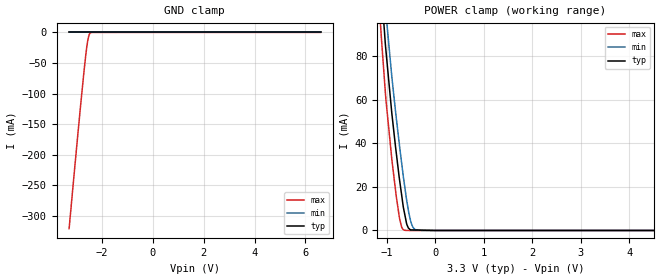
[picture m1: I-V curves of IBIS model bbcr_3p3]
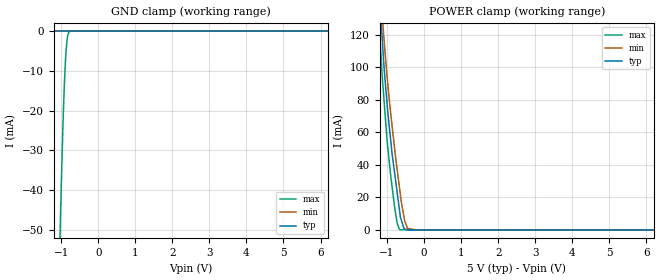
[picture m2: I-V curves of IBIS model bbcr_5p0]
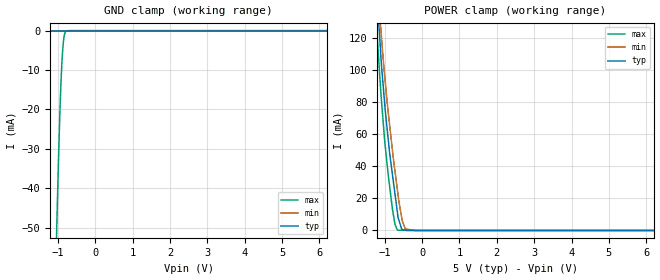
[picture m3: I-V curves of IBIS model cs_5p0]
|Texas Instruments Incorporated
|18 Bit 500KSPS Parallel ADC
| Marketing part#   Digital Voltage Range   Package-type   #pins
| ADS8383IBPFBT   2.95V - 5.25V   TQFP   48
| ADS8383IBPFBTG4   2.95V - 5.25V   TQFP   48
| ADS8383IPFBT   2.95V - 5.25V   TQFP   48
| ADS8383IPFBTG4   2.95V - 5.25V   TQFP   48
[IBIS Ver]   3.2
[File name]   ads8383.ibs
|SIMDE Ver   V3.0 - 201101 - RHL4 - Build 457
[File Rev]   1.1
[Date]   11/11/2011
[Source]
| Texas Instruments Incorporated.
| Analog-eLab Design Center, HPA
| 12500 TI Blvd
| Dallas, TX -75243
| e-mail: elab_scm_ibis@list.ti.com
[Notes]   Revision History:
| Rev 1.1: 11/11/2011
| - Model generated from simulations in TISPICE
| - Model matched to SPICE simulation
| - C_comp although listed in numerical order of value are
|   obtained from varying PVT conditions. For PVT conditions for
|   each specific value refer the buffer description under
|   respective [Model]. IBIS model user is responsible for using
|   appropriate C_comp to simulate for Signal Integrity.
| - Model names with a trailing _5 contains the model for
|   5V [4.75V and 5.25V].
| - Model names with a trailing _3p3 contains the model for
|   3.3V [3V and 3.6V].
[Disclaimer]
| This model is designed as an aid for customers of Texas Instruments.
| TI and its licensors and suppliers make no warranties, either expressed
| or implied, with respect to this  model, including the warranties of
| merchantability or fitness for a particular purpose. The model is
| provided solely on an "as is" basis. The entire risk as to its quality
| and performance is with the customer.
[Copyright]
 (C) Copyright 2011 Texas Instruments Incorporated.All rights reserved.
|   ADS8383PFB
[Component]   ADS8383PFB
[Manufacturer]   TI
[Package]   |48 TQFP  -  PFB package
|   typ   min   max
R_pkg   0.087796   0.08287   0.10031
L_pkg   2.915612nH   2.61503nH   3.79551nH
C_pkg   0.471017pF   0.40218pF   0.58411pF
[Pin]  signal_name   model_name   R_pin   L_pin   C_pin
1   REFIN   TERM   0.10010   3.79551nH  0.57733pF
2   NC   NC   0.09197   3.05397nH  0.50922pF
3   NC   NC   0.08751   2.91787nH  0.48805pF
4   +VA   POWER   0.08536   2.88283nH  0.48088pF
5   AGND   GND   0.08494   2.68463nH  0.43457pF
6   +IN   TERM   0.08529   2.66218nH  0.40388pF
7   -IN   TERM   0.08477   2.65050nH  0.40398pF
8   AGND   GND   0.08402   2.66577nH  0.43614pF
9   +VA   POWER   0.08491   2.87617nH  0.48351pF
10   +VA   POWER   0.08836   2.93642nH  0.49009pF
11   AGND   GND   0.09080   3.03060nH  0.51172pF
12   AGND   GND   0.10050   3.79783nH  0.58722pF
13   +VA   POWER   0.09984   3.80136nH  0.57430pF
14   AGND   GND   0.09184   3.06007nH  0.50608pF
15   AGND   GND   0.08798   2.93541nH  0.48558pF
16   DB17   DB   0.08570   2.89372nH  0.48372pF
17   DB16   DB   0.08388   2.66997nH  0.43641pF
18   DB15   DB   0.08343   2.63103nH  0.40274pF
19   DB14   DB   0.08310   2.62211nH  0.40279pF
20   DB13   DB   0.08287   2.64801nH  0.43550pF
21   DB12   DB   0.08400   2.86018nH  0.48130pF
22   DB11   DB   0.08636   2.90203nH  0.48479pF
23   DB10   DB   0.09049   3.02875nH  0.50816pF
24   +VBD   POWER   0.09815   3.75628nH  0.57908pF
25   BDGND   GND   0.09823   3.76461nH  0.57325pF
26   DB9   DB   0.09338   3.08747nH  0.50871pF
27   DB8   DB   0.08903   2.95227nH  0.48968pF
28   DB7   DB   0.08642   2.90683nH  0.48351pF
29   DB6   DB   0.08500   2.68753nH  0.43735pF
30   DB5   DB   0.08491   2.65538nH  0.40456pF
31   DB4   DB   0.08489   2.65260nH  0.40489pF
32   DB3   DB   0.08497   2.68317nH  0.43773pF
33   DB2   DB   0.08639   2.90287nH  0.48281pF
34   DB1   DB   0.08893   2.94342nH  0.48973pF
35   DB0   DB   0.09324   3.07400nH  0.51329pF
36   BUSY   BUSY   0.10031   3.78743nH  0.58411pF
37   +VBD   POWER   0.09816   3.75870nH  0.57356pF
38   BUS18/_16   BBCR   0.09050   3.02494nH  0.50569pF
39   BYTE   BBCR   0.08638   2.89432nH  0.48541pF
40   _CONVST   BBCR   0.08400   2.85234nH  0.48080pF
41   _RD   BBCR   0.08288   2.64046nH  0.43471pF
42   _CS   CS   0.08311   2.61503nH  0.40218pF
43   +VA   POWER   0.08344   2.61976nH  0.40287pF
44   AGND   GND   0.08386   2.65850nH  0.43615pF
45   AGND   GND   0.08552   2.88190nH  0.48159pF
46   +VA   POWER   0.08742   2.91318nH  0.48615pF
47   REFM   TERM   0.09183   3.04637nH  0.51100pF
48   REFM   TERM   0.09993   3.78233nH  0.58273pF
|   Model Selectors
[Model Selector] BBCR
bbcr_3p3   3.3V   digital input
bbcr_5p0   5V   digital input
[Model Selector] CS
cs_3p3   3.3V   digital input
cs_5p0   5V   digital input
[Model Selector] BUSY
busy_3p3   3.3V   digital output
busy_5p0   5V   digital output
[Model Selector] DB
dbp_3p3   3.3V   digital 3-state
dbp_5p0   5V   digital 3-state
[Model Selector] TERM
term_3p3   3.3V   nominal termination
term_5p0   5V   nominal termination
[Model] term_5p0
Model_type Terminator
C_comp   1.0e-20F  1.0e-20F  1.0e-20F
|   typ   min   max
[Voltage Range]   5V   4.75V   5.25V
[POWER Clamp Reference]   5V   4.75V   5.25V
[GND Clamp Reference]   0V   0V   0V
|Ambient Temperature   25   85   -40
|Junction Temperature
[Temperature Range]   35   95   -40
[Model] term_3p3
Model_type Terminator
C_comp   1.0e-20F  1.0e-20F  1.0e-20F
|   typ   min   max
[Voltage Range]   3.3V   3V   3.6V
[POWER Clamp Reference]   3.3V   3V   3.6V
[GND Clamp Reference]   0V   0V   0V
|Ambient Temperature   25   85   -40
|Junction Temperature
[Temperature Range]   35   95   -40
| Models and submodels in the file (10): bbcr_3p3 (Input), bbcr_5p0 (Input), cs_3p3 (Input), cs_5p0 (Input), busy_3p3 (Output), busy_5p0 (Output), dbp_3p3 (3-state), dbp_5p0 (3-state), term_5p0 (Terminator), term_3p3 (Terminator)
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|   bbcr_3p3 Model
[Model]   bbcr_3p3
Model_type   Input
Vinl = 0.8
Vinh = 2.3
|   typ   min   max
|   (nom PVT)   (fast PVT)   (slow PVT)
|C_comp from frequency sweep method (F=500KHz)
|Average
|C_comp   1.695e-12   1.582e-12   1.872e-12
|C_comp from LC tank measurement(L=1nH)
|Average
|Resonant Frequency(Hz)   4.320e+09   4.570e+09   4.100e+09
C_comp   1.359e-12   1.214e-12   1.508e-12
[Model spec]
|subparameter
Vinl   0.8   0.8   0.8
Vinh   2.3   2.0   2.6
| Where nom  PVT is Nominal Process, 3.3V, 35C
|   Fast PVT is Strong Process,  3.6V, -40C
|   Slow PVT is Weak Process,   3V, 95C
[Voltage Range]   3.3   3   3.6
|Ambient Temperature   25   85   -40
|Junction Temperature
[Temperature Range]   35   95   -40
[Power Clamp Reference]   3.3   3   3.6
[GND Clamp Reference]   0   0   0
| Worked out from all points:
|   POWER clamp passes 1 mA (typ) near -0.55 V on its own axis
[GND Clamp]
|   Voltage   I(typ)   I(min)   I(max)
-3.3V     0A         0A         -320.7mA
-2.945V   0A         0A         -161.8mA
-2.826V   0A         0A         -110.3mA
-2.722V   0A         0A         -66.93mA
-2.632V   0A         0A         -32.94mA
-2.581V   0A         0A         -17.4mA
-2.52V    0A         0A         -5.192mA
-2.473V   0A         0A         -1.113mA
-2.412V   0A         0A         -67.52uA
6.6V      0A         0A         0A
[POWER Clamp]
|   Voltage   I(typ)   I(min)   I(max)
-3.3V     1.065A     1.069A     1.058A
-1.148V   121.8mA    138.2mA    100.8mA
-1.12V    112.9mA    128.9mA    90.76mA
-1.03V    85.2mA     102.5mA    63.02mA
-1.015V   81.78mA    98.96mA    59.18mA
-806.4mV  35.7mA     51.92mA    15.75mA
-738mV    23.21mA    38.69mA    5.486mA
-637.2mV  8.056mA    21.08mA    124.8uA
-587.4mV  2.72mA     13.29mA    13.69uA
-504mV    265.4uA    3.789mA    169.8nA
-285mV    149.3uA    6.628uA    0A
6.6V      0A         0A         0A
|   bbcr_5p0 Model
[Model]   bbcr_5p0
Model_type   Input
Vinl = 0.8
Vinh = 4
|   typ   min   max
|   (nom PVT)   (fast PVT)   (slow PVT)
|C_comp from frequency sweep method (F=500KHz)
|Average
|C_comp   1.617e-12   1.527e-12   1.728e-12
|C_comp from LC tank measurement(L=1nH)
|Average
|Resonant Frequency(Hz)   4.440e+09   4.680e+09   4.240e+09
C_comp   1.286e-12   1.158e-12   1.410e-12
[Model spec]
|subparameter
Vinl   0.8   0.8   0.8
Vinh   4.0   3.75   4.25
| Where nom  PVT is Nominal Process, 5V, 35C
|   Fast PVT is Strong Process,  5.25V, -40C
|   Slow PVT is Weak Process,   4.75V, 95C
[Voltage Range]   5   4.75   5.25
|Ambient Temperature   25   85   -40
|Junction Temperature
[Temperature Range]   35   95   -40
[Power Clamp Reference]   5   4.75   5.25
[GND Clamp Reference]   0   0   0
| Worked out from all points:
|   POWER clamp passes 1 mA (typ) near -0.54 V on its own axis
[GND Clamp]
|   Voltage   I(typ)   I(min)   I(max)
-5V       0A         0A         -1.868A
-1.055V   0A         0A         -60.42mA
-1.024V   0A         0A         -48.22mA
-997.5mV  0A         0A         -38.53mA
-955.5mV  0A         0A         -24.41mA
-918.7mV  0A         0A         -14.26mA
-887.2mV  0A         0A         -7.806mA
-866.2mV  0A         0A         -4.706mA
-840mV    0A         0A         -2.1mA
-803.3mV  0A         0A         -473.2uA
-761.2mV  0A         0A         -65.11uA
10V       0A         0A         0A
[POWER Clamp]
|   Voltage   I(typ)   I(min)   I(max)
-5V       1.847A     1.85A      1.843A
-1.202V   143mA      156.3mA    121.8mA
-1.134V   118.7mA    133.8mA    95.73mA
-1.102V   107.3mA    123.4mA    86.04mA
-1.003V   78.52mA    95.39mA    55.99mA
-903mV    55.52mA    72.05mA    33.79mA
-724.5mV  22.65mA    36.66mA    3.969mA
-640.5mV  8.033mA    21.75mA    146.3uA
-527.2mV  588.5uA    5.844mA    120.4uA
-446.5mV  169.9uA    938.2uA    102uA
-190mV    0A         331.6nA    43.4uA
10V       0A         0A         0A
|   cs_5p0 Model
[Model]   cs_5p0
Model_type   Input
Vinl = 0.8
Vinh = 4
|   typ   min   max
|   (nom PVT)   (fast PVT)   (slow PVT)
|C_comp from frequency sweep method (F=500KHz)
|Average
|C_comp   1.617e-12   1.527e-12   1.728e-12
|C_comp from LC tank measurement(L=1nH)
|Average
|Resonant Frequency(Hz)   4.440e+09   4.680e+09   4.240e+09
C_comp   1.286e-12   1.158e-12   1.410e-12
[Model spec]
|subparameter
Vinl   0.8   0.8   0.8
Vinh   4.0   3.75   4.25
| Where nom  PVT is Nominal Process, 5V, 35C
|   Fast PVT is Strong Process,  5.25V, -40C
|   Slow PVT is Weak Process,   4.75V, 95C
[Voltage Range]   5   4.75   5.25
|Ambient Temperature   25   85   -40
|Junction Temperature
[Temperature Range]   35   95   -40
[Power Clamp Reference]   5   4.75   5.25
[GND Clamp Reference]   0   0   0
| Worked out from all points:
|   POWER clamp passes 1 mA (typ) near -0.54 V on its own axis
[GND Clamp]
|   Voltage   I(typ)   I(min)   I(max)
-5V       0A         0A         -1.887A
-1.055V   0A         0A         -61.13mA
-1.024V   0A         0A         -48.8mA
-997.5mV  0A         0A         -39mA
-955.5mV  0A         0A         -24.71mA
-918.7mV  0A         0A         -14.44mA
-887.2mV  0A         0A         -7.896mA
-866.2mV  0A         0A         -4.751mA
-840mV    0A         0A         -2.113mA
-803.3mV  0A         0A         -474.1uA
-761.2mV  0A         0A         -65.13uA
10V       0A         0A         0A
[POWER Clamp]
|   Voltage   I(typ)   I(min)   I(max)
-5V       1.868A     1.87A      1.863A
-1.302V   181.5mA    196mA      162.6mA
-1.197V   143.7mA    157.3mA    120.7mA
-1.134V   120.9mA    136.3mA    97.41mA
-1.097V   107.5mA    124.2mA    84.81mA
-992.2mV  77.12mA    94.59mA    54.43mA
-792.7mV  35.19mA    50.41mA    13.69mA
-640.5mV  8.137mA    22.11mA    146.4uA
-527.2mV  589.9uA    5.903mA    120.5uA
-446.5mV  170.3uA    940.6uA    102.1uA
-190mV    0A         331.6nA    43.43uA
10V       0A         0A         0A
